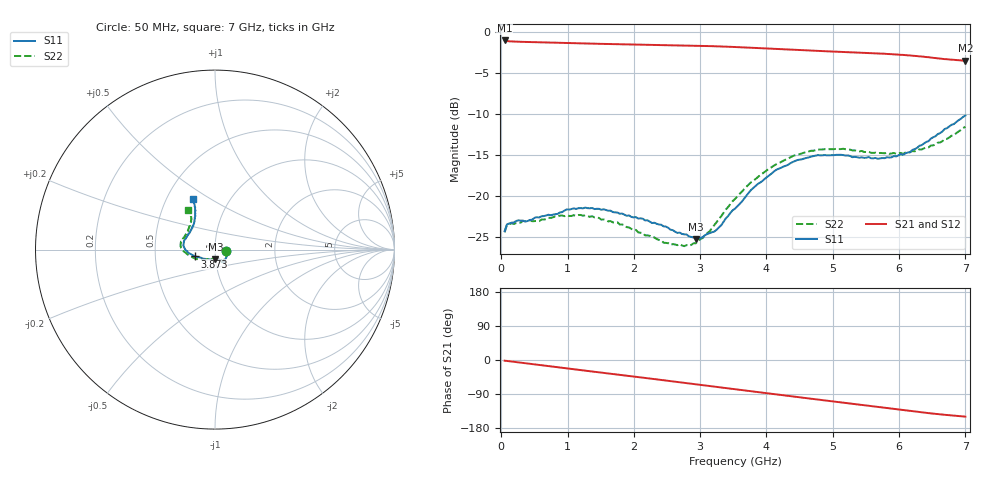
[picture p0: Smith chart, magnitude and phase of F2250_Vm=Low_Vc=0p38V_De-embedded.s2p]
! Integrated Device Technology
! Corporate Headquarters
! 6024 Silver Creek Valley Road
! San Jose, CA 95138  USA
! Phone:  1-408-284-8200
! Toll Free:  1-800-223-1366
! Webpage:  http://www.idt.com/
! Timing and RF Division
! 515 Groton Road, Suite 102
! Westford, MA 01886-6024
! Device:  F2250
! Description: Voltage Variable RF Attenuator
! Frequency:  50.0 -  6000.00 MHz
! Package:  3x3 mm Thin QFN Plastic Package: 16 pin
! Ports:  2 RF, 3 DC
!  Pin  1  = GND
!  Pin  2  = NC
!  Pin  3  = RF1  = Port 1
!  Pin  4  = NC
!  Pin  5  = GND
!  Pin  6  = GND
!  Pin  7  = GND
!  Pin  8  = GND
!  Pin  9  = NC
!  Pin 10  = RF2  = Port 2
!  Pin 11  = NC
!  Pin 12  = GND
!  Pin 13  = GND
!  Pin 14  = VCNTRL
!  Pin 15  = VDD
!  Pin 16  = VMODE
! Vcntrl:  0.380 Volts
! Vmode:  +0.000 Volts
! Vdd:  +3.30  Volts
! Current:  1.121 mA
! Data:  The device was measured on a the F2250 evaluation board which has
!  individual transmission lines to the RF pins.  Data was collected
!  using a calibrated network analyzer.  The evaluation board was
!  de-embedded using a TRL calibration technique.
!  The reference plane is the edge of the package pin.
! Misc:  SN 10
!  Action Tracker AT0258
! Date Measured:  2014-11-26
! Date:  2015-10-15  MJV
! Note:
!  Integrated Device Technology supplies this data as a sample of measured
!  data at the package pin for this product.  Your particular data for this
!  product may vary.
!  Data was taken at 25 degrees C.
!  Integrated Device Technology reserves the right to change this data at anytime.
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# GHz S dB R 50
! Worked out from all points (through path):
!   201 points, 50 MHz to 7 GHz, reference 50 ohm
!   highest |S21| = -0.98 dB at 50 MHz (marker M1); lowest = -3.5 dB at 7 GHz (marker M2)
!   group delay of S21, straight-line fit = 60 ps
!   lowest |S11| = -25.2 dB at 2.934 GHz (marker M3), VSWR 1.12, Z = 49.9 - j5.49 ohm
!   |S11| at or under -10 dB: start of sweep to end of sweep
!   |S22| runs from -26.1 to -11.5 dB; largest |S21 - S12| = 0.00034
!   S11 on the Smith chart (normalised r, x): 50 MHz: 1.13, -0.02; 3.873 GHz: 0.80, -0.06; 7 GHz: 0.67, +0.42
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0.05  -24.26 -8.9  -0.98 -1.8  -0.98 -1.8  -24.40 -9.5
0.08475  -23.44 -8.8  -1.06 -2.5  -1.05 -2.5  -23.53 -8.8
0.15425  -23.23 -11.0  -1.10 -4.0  -1.10 -4.0  -23.30 -10.6
0.57125  -22.59 -28.3  -1.20 -13.1  -1.20 -13.1  -23.04 -29.4
0.71025  -22.25 -36.1  -1.23 -16.2  -1.23 -16.2  -22.62 -37.3
1.2315  -21.48 -53.4  -1.35 -27.4  -1.34 -27.4  -22.37 -58.2
1.75275  -21.99 -60.0  -1.44 -38.4  -1.44 -38.4  -23.18 -65.9
2.37825  -23.45 -61.2  -1.53 -51.8  -1.53 -51.8  -25.33 -69.0
2.552  -24.08 -65.0  -1.55 -55.6  -1.55 -55.6  -25.94 -74.7
2.83  -24.91 -79.2  -1.60 -61.7  -1.60 -61.7  -26.06 -92.9
2.93425  -25.21 -87.6  -1.62 -64.0  -1.62 -64.0  -25.75 -101.3
3.21225  -24.32 -116.5  -1.69 -70.2  -1.69 -70.2  -23.52 -126.3
3.525  -21.52 -144.2  -1.78 -77.1  -1.78 -77.1  -20.33 -145.2
3.8725  -18.48 -161.4  -1.91 -84.8  -1.91 -84.8  -17.64 -160.6
4.1505  -16.76 -171.5  -2.02 -90.9  -2.02 -90.9  -16.08 -170.7
4.4285  -15.71 -179.3  -2.13 -96.9  -2.13 -96.9  -15.00 -177.9
4.7065  -15.11 173.9  -2.23 -102.9  -2.24 -102.9  -14.44 176.1
5.15825  -14.97 163.1  -2.39 -112.6  -2.39 -112.6  -14.20 166.8
5.85325  -15.28 139.8  -2.64 -127.6  -2.64 -127.6  -14.81 151.6
6.166  -14.59 128.7  -2.81 -134.4  -2.81 -134.4  -14.64 142.7
6.444  -13.28 120.2  -3.02 -140.2  -3.02 -140.2  -14.04 133.3
7  -10.15 113.7  -3.46 -149.5  -3.46 -149.5  -11.51 123.8
